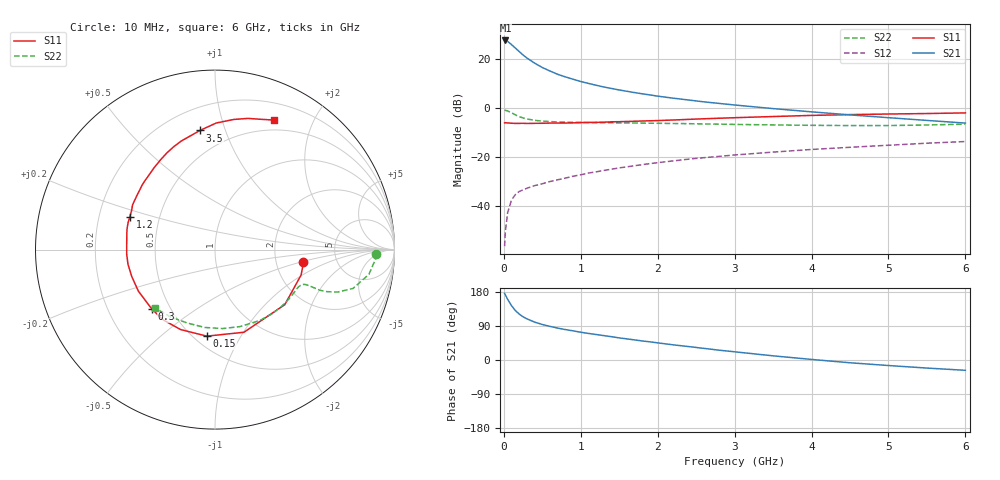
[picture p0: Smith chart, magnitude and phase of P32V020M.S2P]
! SIEMENS Small Signal Semiconductors
! BFP181
! Si NPN RF Bipolar Junction Transistor in SOT143
! VCE = 2 V  IC = 20 mA
! Common Emitter S-Parameters:  March  1996
# GHz  S  MA  R  50
!  f  S11  S21  S12  S22
! GHz  MAG  ANG  MAG  ANG  MAG  ANG  MAG  ANG
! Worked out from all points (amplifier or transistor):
!   36 points, 10 MHz to 6 GHz, reference 50 ohm
!   highest |S21| = 27.6 dB at 20 MHz (marker M1)
!   |S21| within 3 dB of that: start of sweep to 146 MHz
!   unconditionally stable (mu >= 1): start of sweep to 19.87 MHz; 334 MHz to end of sweep
!   at 250 MHz: K = 0.83, MSG = 27.6 dB, |S12| = -33.5 dB
!   at 1.4 GHz: K = 1.76, MAG = 11.5 dB, |S12| = -25.0 dB
!   at 6 GHz: K = 1.33, MAG = 0.3 dB, |S12| = -13.7 dB
!   S11 on the Smith chart (normalised r, x): 10 MHz: 2.87, -0.54; 150 MHz: 0.58, -0.73; 300 MHz: 0.40, -0.34; 1.2 GHz: 0.34, +0.17; 3.5 GHz: 0.34, +0.82; 6 GHz: 0.38, +1.49
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0.01  0.498 -8.2  24 175.8  0.0015 79.0  0.8996 -1.6
0.02  0.5003 -16.4  24 172.0  0.003 88.3  0.8949 -3.6
0.05  0.4953 -38.3  22.93 159.9  0.0073 75.0  0.8687 -9.1
0.1  0.488 -70.7  19.76 143.3  0.0132 61.9  0.7992 -15.7
0.15  0.4843 -95.4  16.77 130.4  0.017 55.3  0.7229 -19.1
0.2  0.4851 -113.3  14.22 121.1  0.0197 52.1  0.6663 -20.6
0.25  0.4863 -126.4  12.12 114.0  0.0212 49.6  0.6259 -21.2
0.3  0.4833 -136.7  10.51 108.6  0.0229 49.0  0.5967 -21.1
0.4  0.4856 -151.5  8.257 100.0  0.0259 49.0  0.5601 -21.0
0.5  0.4875 -162.1  6.717 93.7  0.0283 49.6  0.5397 -21.1
0.6  0.4916 -170.4  5.697 88.7  0.0314 51.4  0.5276 -21.6
0.7  0.4926 -177.0  4.879 84.2  0.0341 53.0  0.5188 -22.2
0.8  0.4926 177.4  4.324 80.3  0.0369 54.1  0.5149 -23.0
1.1  0.507 162.9  3.182 70.1  0.0468 55.6  0.5035 -26.5
1.2  0.5086 158.8  2.915 67.3  0.0496 56.0  0.5022 -28.0
1.6  0.5302 144.6  2.195 55.7  0.0628 56.3  0.4946 -34.0
2.2  0.5683 126.7  1.589 40.1  0.0829 54.0  0.4823 -44.6
2.8  0.6178 111.8  1.24 25.9  0.1027 50.3  0.4683 -56.5
3.5  0.669 97.2  0.972 11.0  0.1255 45.6  0.451 -72.1
4.5  0.7322 81.9  0.723 -7.3  0.1574 37.1  0.4375 -97.5
5.5  0.7704 70.4  0.557 -21.3  0.1907 28.8  0.4496 -123.6
6  0.7937 65.4  0.492 -27.2  0.2064 24.0  0.4675 -136.0
